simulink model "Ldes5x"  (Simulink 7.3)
settings: Solver=ode45  StartTime=0.0  StopTime=10.0  RelTol=1e-3
undefined symbols (not defined in the file or in its folder): Als, Bls, Cls, Dls, Kmix

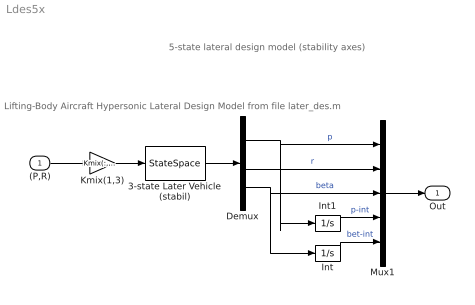
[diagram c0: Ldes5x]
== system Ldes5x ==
  note: 5-state lateral design model (stability axes)
  note: Lifting-Body Aircraft Hypersonic Lateral Design Model from file later_des.m
  (P,R) : Inport  OutDataType=sfix(16)  OutScaling=2^0
  3-state Later Vehicle (stabil) : StateSpace  A=Als  B=Bls  C=Cls  D=Dls
  Demux : Demux  Outputs=3
  Int : Integrator
  Int1 : Integrator
  Kmix(1,3) : Gain  Gain=Kmix(:,[1,3])  Multiplication=Matrix(K*u)  ParameterDataType=sfix(16)  ParameterScaling=2^0  OutDataType=sfix(16)  OutScaling=2^0
  Mux1 : Mux  Inputs=5
  Out : Outport  OutDataType=sfix(16)  OutScaling=2^0
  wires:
  3-state Later Vehicle (stabil)/1 -> Demux/1
  Demux/1 -> Mux1/1, Int1/1  "p"
  Demux/2 -> Mux1/2  "r"
  Mux1/1 -> Out/1
  (P,R)/1 -> Kmix(1,3)/1
  Demux/3 -> Int/1, Mux1/3  "beta"
  Int/1 -> Mux1/5  "bet-int"
  Int1/1 -> Mux1/4  "p-int"
  Kmix(1,3)/1 -> 3-state Later Vehicle (stabil)/1
